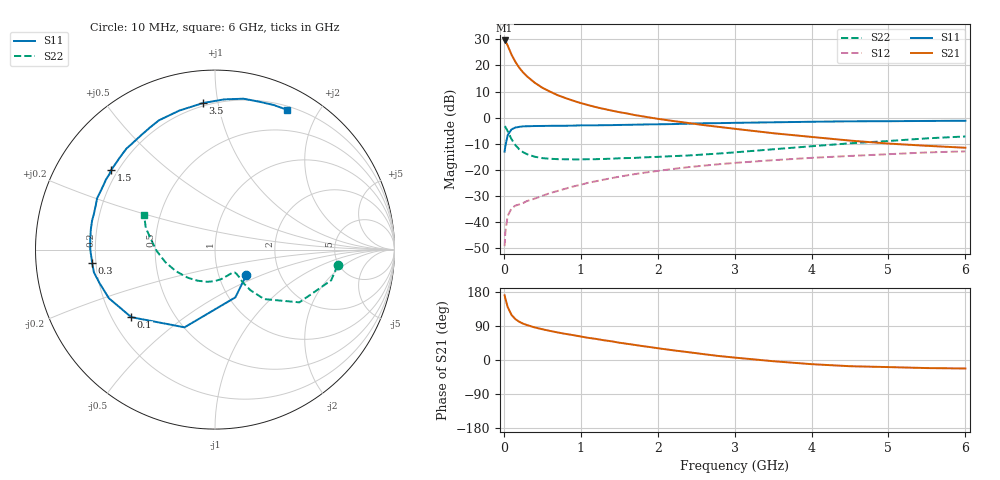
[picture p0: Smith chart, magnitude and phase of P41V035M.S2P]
! SIEMENS Small Signal Semiconductors
! BFP182
! Si NPN RF Bipolar Junction Transistor in SOT143
! VCE = 1 V  IC = 35 mA
! Common Emitter S-Parameters:  March  1996
# GHz  S  MA  R  50
!  f  S11  S21  S12  S22
! GHz  MAG  ANG  MAG  ANG  MAG  ANG  MAG  ANG
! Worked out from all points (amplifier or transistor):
!   36 points, 10 MHz to 6 GHz, reference 50 ohm
!   highest |S21| = 29.6 dB at 10 MHz (marker M1)
!   |S21| within 3 dB of that: start of sweep to 64.97 MHz
!   unconditionally stable (mu >= 1): start of sweep to 32.12 MHz; 150.1 MHz to end of sweep
!   at 250 MHz: K = 1.39, MAG = 21.2 dB, |S12| = -32.6 dB
!   at 1.4 GHz: K = 2.36, MAG = 6.4 dB, |S12| = -23.1 dB
!   at 6 GHz: K = 1.81, MAG = -4.5 dB, |S12| = -12.8 dB
!   S11 on the Smith chart (normalised r, x): 10 MHz: 1.35, -0.41; 100 MHz: 0.28, -0.33; 300 MHz: 0.19, -0.05; 1.5 GHz: 0.17, +0.33; 3.5 GHz: 0.18, +0.90; 6 GHz: 0.24, +1.61
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0.01  0.2251 -39.2  30.12 170.7  0.0035 70.6  0.6887 -7.3
0.02  0.2893 -66.9  29.37 162.0  0.0066 65.1  0.6695 -14.8
0.05  0.4651 -111.4  24.04 139.8  0.0133 58.2  0.5546 -32.0
0.1  0.5995 -141.1  16.11 118.9  0.0185 41.8  0.3887 -45.2
0.15  0.6504 -155.4  11.74 107.9  0.0209 38.7  0.3002 -48.9
0.2  0.6696 -163.7  9.075 100.9  0.022 39.2  0.2499 -49.6
0.25  0.6865 -169.4  7.373 95.9  0.0234 41.0  0.2198 -49.4
0.3  0.6883 -173.6  6.212 92.3  0.0255 42.3  0.2013 -48.7
0.4  0.6949 -180.0  4.702 86.0  0.0284 45.8  0.1802 -48.4
0.5  0.6977 174.8  3.757 81.2  0.0321 48.8  0.169 -49.1
0.6  0.7009 170.7  3.165 76.8  0.0363 51.4  0.1646 -50.5
0.7  0.7037 166.8  2.705 72.7  0.0398 53.2  0.1616 -52.4
0.8  0.7035 163.4  2.385 69.0  0.044 54.5  0.1606 -54.9
1.1  0.7154 153.5  1.741 58.4  0.0572 55.8  0.1612 -64.3
1.5  0.7293 142.3  1.281 45.7  0.0746 55.1  0.1679 -77.6
1.8  0.7425 133.7  1.067 36.8  0.088 53.3  0.1742 -88.7
2.2  0.7577 123.3  0.868 25.6  0.105 49.6  0.1848 -103.7
2.8  0.7903 108.7  0.668 10.4  0.1294 43.2  0.2072 -127.2
3.5  0.8192 94.7  0.507 -3.2  0.1544 35.5  0.2495 -151.4
4.5  0.8556 79.3  0.366 -16.4  0.1861 24.8  0.3248 -178.6
5.5  0.8693 67.9  0.291 -21.3  0.2172 14.4  0.404 162.6
6  0.8763 62.8  0.267 -22.4  0.2278 8.6  0.4393 154.1
